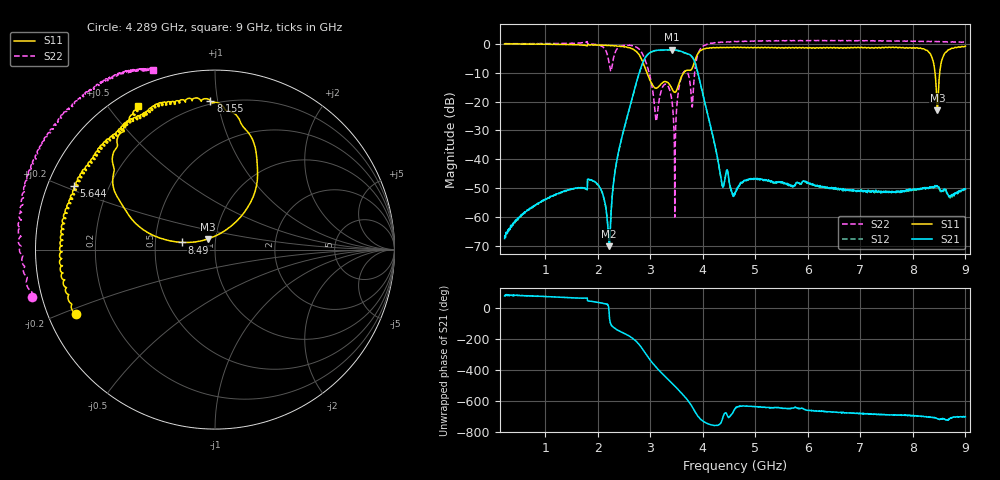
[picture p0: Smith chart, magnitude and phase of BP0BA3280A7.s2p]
!Agilent Technologies,E8358A,US41080443,A.07.50.56
!Agilent E8358A: A.07.50.56
!Date: Friday, July 21, 2017 20:13:26
!Correction: S11(Full 2 Port(1,2))
!S21(Full 2 Port(1,2))
!S12(Full 2 Port(1,2))
!S22(Full 2 Port(1,2))
!S2P File: Measurements: S11, S21, S12, S22:
# Hz S  dB  R 50
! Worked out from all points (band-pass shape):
!   1601 points, 225 MHz to 9 GHz, reference 50 ohm
!   highest |S21| = -2.10 dB at 3.411 GHz (marker M1); lowest = -70.0 dB at 2.216 GHz (marker M2)
!   |S21| within 3 dB of the highest: 2.894 GHz to 3.818 GHz (923.9 MHz wide, 27.5 % of centre)
!   lowest |S11| = -23.0 dB at 8.468 GHz (marker M3), VSWR 1.15, Z = 46 + j5.52 ohm
!   |S11| at or under -10 dB: 2.933 GHz to 3.637 GHz (703.8 MHz wide, 21.4 % of centre); 8.421 GHz to 8.511 GHz (89.74 MHz wide, 1.06 % of centre)
!   |S22| runs from -60.0 to 1.1 dB; largest |S21 - S12| = 0.014
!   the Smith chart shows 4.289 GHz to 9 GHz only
!   S11 on the Smith chart (normalised r, x): 4.289 GHz: 0.08, -0.22; 5.644 GHz: 0.08, +0.21; 8.155 GHz: 0.18, +0.95; 8.49 GHz: 0.69, +0.06; 9 GHz: 0.07, +0.60
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2.25e8  -0.05 177.3  -67.38 77.2  -66.84 84.4  0.01 176.1
1.689328e9  -0.43 147.4  -49.78 62.8  -49.81 62.9  0.31 159.5
2.045812e9  -0.53 142.9  -49.92 32.3  -50.02 32.6  -0.66 94.0
2.215828e9  -0.56 133.7  -70.02 -31.3  -69.95 -30.8  -6.83 5.0
2.380359e9  -0.87 121.5  -38.63 -144.9  -38.70 -145.4  -1.56 160.1
2.791688e9  -3.92 24.1  -9.84 120.6  -9.95 120.9  -1.94 75.2
2.939766e9  -10.32 -77.5  -3.91 49.5  -4.00 49.3  -7.69 37.2
3.153656e9  -14.92 -136.9  -2.20 -39.8  -2.32 -40.3  -21.25 -149.1
3.411422e9  -15.54 -152.1  -2.10 -126.3  -2.22 -126.8  -19.77 117.7
3.47175e9  -16.82 -131.5  -2.16 -147.1  -2.27 -147.7  -38.00 -84.7
3.592406e9  -11.45 -107.1  -2.70 169.4  -2.80 168.8  -11.54 -122.4
3.745969e9  -9.20 -115.3  -3.73 107.4  -3.84 106.9  -12.33 -171.0
3.959859e9  -2.37 -121.1  -14.27 -0.7  -14.34 -1.0  -1.61 -118.6
4.288922e9  -1.39 -155.2  -40.44 -38.7  -40.50 -38.7  0.47 -165.6
4.6125e9  -1.31 -171.3  -51.65 68.6  -51.80 67.6  0.80 177.1
5.643562e9  -1.31 155.8  -48.93 70.7  -48.62 67.2  1.05 148.6
6.076828e9  -1.51 145.0  -48.60 56.8  -48.83 55.9  1.05 139.5
7.541156e9  -1.19 112.6  -51.32 28.4  -51.29 29.0  0.91 119.6
8.155406e9  -1.61 91.8  -50.07 19.3  -50.16 20.5  0.84 115.2
8.468016e9  -23.01 122.5  -49.25 3.8  -49.24 2.5  0.70 113.1
8.489953e9  -14.58 167.6  -49.69 0.8  -49.72 -1.8  0.77 112.8
9e9  -0.86 118.3  -50.33 16.5  -50.08 16.9  0.51 108.9
